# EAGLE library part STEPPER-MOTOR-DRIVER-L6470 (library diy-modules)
Stepper Motor Driver based on L6470 chip More details can be found here: https://www.sparkfun.com/products/retired/10859 L6470 datasheet is available here: www.st.com/resource/en/datasheet/CD00255075.pdf Click here to find device on ebay.com
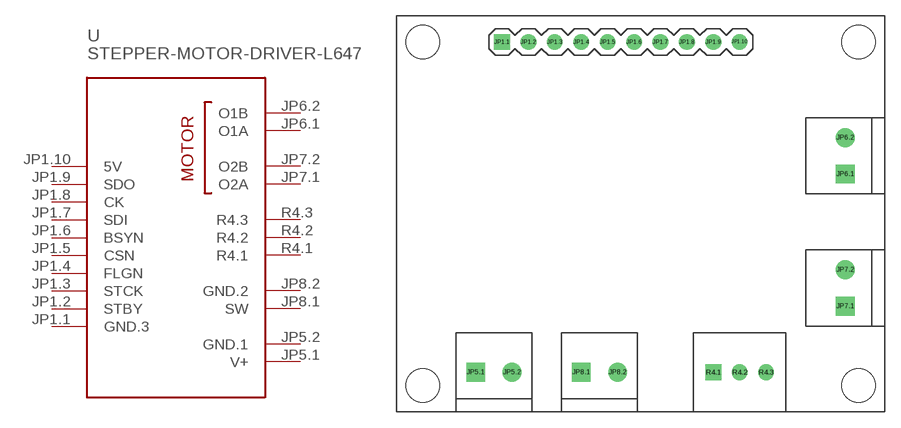
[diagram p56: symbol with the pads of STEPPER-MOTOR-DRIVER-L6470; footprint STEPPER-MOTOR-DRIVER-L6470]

Designator prefix -

## STEPPER-MOTOR-DRIVER-L6470  [STEPPER-MOTOR-DRIVER-L6470]
JP1.1  GND.3  pwr
JP1.2  STBY
JP1.3  STCK
JP1.4  FLGN
JP1.5  CSN
JP1.6  BSYN
JP1.7  SDI
JP1.8  CK
JP1.9  SDO
JP1.10  5V  pwr
JP5.1  V+  pwr
JP5.2  GND.1  pwr
JP6.1  O1A  out
JP6.2  O1B  out
JP7.1  O2A  out
JP7.2  O2B  out
JP8.1  SW
JP8.2  GND.2
R4.1  R4.1  pas
R4.2  R4.2  pas
R4.3  R4.3  pas

## Footprint STEPPER-MOTOR-DRIVER-L6470 (pad centres in mm)
Stepper Motor Driver based on L6470 chip
drill 1 square: JP1.1 -13.335,16.51; R4.1 6.985,-15.24
drill 1: JP1.2 -10.795,16.51; JP1.3 -8.255,16.51; JP1.4 -5.715,16.51; JP1.5 -3.175,16.51; JP1.6 -0.635,16.51; JP1.7 1.905,16.51; JP1.8 4.445,16.51; JP1.9 6.985,16.51; JP1.10 9.525,16.51; R4.2 9.525,-15.24; R4.3 12.065,-15.24
drill 1.2 square: JP5.1 -15.875,-15.24; JP6.1 19.685,3.81; JP7.1 19.685,-8.89; JP8.1 -5.715,-15.24
drill 1.2: JP5.2 -12.37,-15.24; JP6.2 19.685,7.315; JP7.2 19.685,-5.385; JP8.2 -2.21,-15.24
hole 3.2 at -20.955,16.51
hole 3.2 at -20.955,-16.51
hole 3.2 at 20.955,16.51
hole 3.2 at 20.955,-16.51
